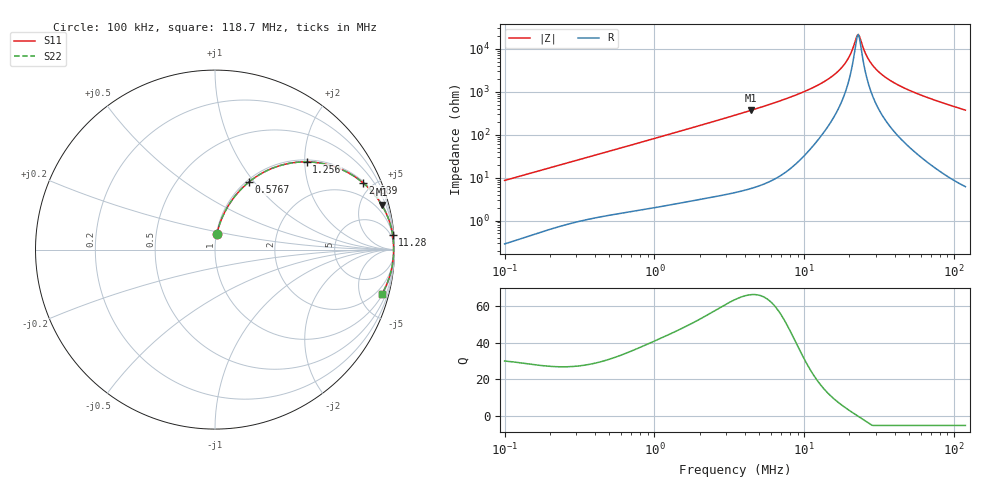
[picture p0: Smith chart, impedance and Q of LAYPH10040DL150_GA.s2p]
! LAYPH10040DL150_GA  S-PARAMETER MODEL  ( General Type )
! Model Generated by TAIYO YUDEN Corporation (http://www.ty-top.com)
! Version 1.0
! TAIYO YUDEN Control No. 180920NI43SB-FBB
! Copyright(c) 2018 TAIYO YUDEN CO.,LTD. All Rights Reserved.
! Product Description (link to TY-COMPAS)
! https://ds.yuden.co.jp/TYCOMPAS/or/detail?pn=LAYPH10040DL150MGA&u=M
! Products Name : Inductors
! Characteristics :
!  Inductance : 15 uH , SRF(min) : -Hz , DC Resistance(max) : 0.052 Ohm
!  Rated Current : Saturation :2.9 A , Temp Rise : 1.6 A (25 degC)
!  Case Size : 10.1 x 10.0 / 0.398 x 0.394 [mm/inch] , Thickness : 4 / 0.157 [mm/inch]
!  (Conditions: Temperature = 25 degC , DC Bias Current/Voltage = 0A / 0V)
! External Node Assignments :
!  1  o---GGG---o  2
! GND o---------o GND
! Frequency Range : 0.1MHz  -  118.695536MHz  [ 402 STEP ]
# MHz S RI R 50
! Freq[MHz].  S11 Real  S11 Imag  S21 Real  S21 Imag  S12 Real  S12 Imag  S22 Real  S22 Imag
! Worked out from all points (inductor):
!   401 points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, 100 kHz to 118.7 MHz, reference 50 ohm
!   read as one part in series: L = 13.6 uH near 103.6 kHz
!   highest Q = 66.1 at 4.414 MHz (marker M1), where L = 13.3 uH
!   self-resonance near 22.49 MHz
!   S11 on the Smith chart (normalised r, x): 100 kHz: 1.01, +0.17; 576.7 kHz: 1.03, +0.95; 1.256 MHz: 1.05, +2.04; 2.689 MHz: 1.07, +4.38; 11.28 MHz: 2, +24; 118.7 MHz: 1.12, -7.42
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0.1  0.0101 0.0845  0.9899 -0.0845  0.9899 -0.0845  0.0101 0.0845
0.327316  0.0767 0.2486  0.9233 -0.2486  0.9233 -0.2486  0.0767 0.2486
0.576664  0.19 0.3773  0.81 -0.3773  0.81 -0.3773  0.19 0.3773
1.07136  0.433 0.4837  0.567 -0.4837  0.567 -0.4837  0.433 0.4837
1.256349  0.5098 0.4888  0.4902 -0.4888  0.4902 -0.4888  0.5098 0.4888
2.689131  0.8236 0.3728  0.1764 -0.3728  0.1764 -0.3728  0.8236 0.3728
3.445222  0.8852 0.3109  0.1148 -0.3109  0.1148 -0.3109  0.8852 0.3109
4.413899  0.928 0.251  0.072 -0.251  0.072 -0.251  0.928 0.251
7.505938  0.9761 0.1432  0.0239 -0.1432  0.0239 -0.1432  0.9761 0.1432
11.27678  0.9899 0.0811  0.0101 -0.0811  0.0101 -0.0811  0.9899 0.0811
14.70538  0.9936 0.048  0.00645 -0.048  0.00645 -0.048  0.9936 0.048
17.55242  0.9948 0.0281  0.00522 -0.0281  0.00522 -0.0281  0.9948 0.0281
19.51882  0.9952 0.0167  0.00482 -0.0167  0.00482 -0.0167  0.9952 0.0167
22.09308  0.9954 0.00353  0.00464 -0.00353  0.00464 -0.00353  0.9954 0.00353
22.88908  0.9954 -0.000206  0.00464 0.000206  0.00464 0.000206  0.9954 -0.000206
23.71377  0.9953 -0.00394  0.00467 0.00394  0.00467 0.00394  0.9953 -0.00394
25.90783  0.9952 -0.0133  0.00484 0.0133  0.00484 0.0133  0.9952 -0.0133
27.80836  0.9949 -0.0209  0.0051 0.0209  0.0051 0.0209  0.9949 -0.0209
31.47588  0.9942 -0.0344  0.00583 0.0344  0.00583 0.0344  0.9942 -0.0344
36.91074  0.9926 -0.0525  0.00736 0.0525  0.00736 0.0525  0.9926 -0.0525
58.47779  0.9826 -0.1136  0.0174 0.1136  0.0174 0.1136  0.9826 -0.1136
118.6955  0.9288 -0.249  0.0712 0.249  0.0712 0.249  0.9288 -0.249
